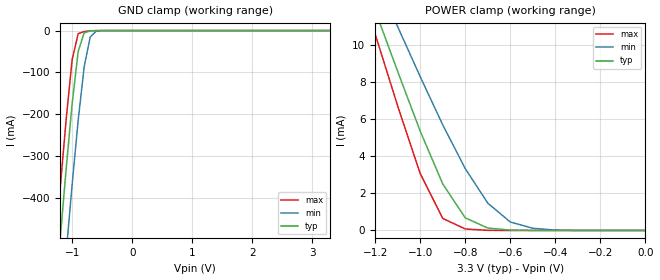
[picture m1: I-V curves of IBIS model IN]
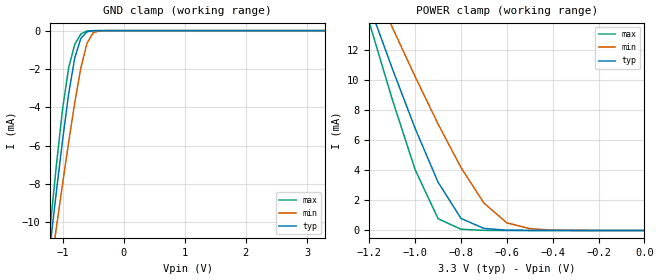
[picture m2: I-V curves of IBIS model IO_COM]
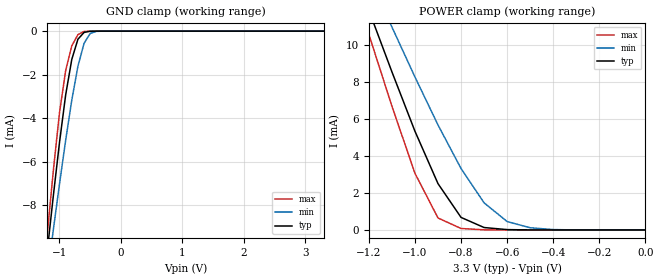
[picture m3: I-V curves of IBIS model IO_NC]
| (C) Copyright DIODES INCORPORATED
| DIODES CORPORATION
| IBIS Model of PI5A23157
| MSOP-10 (U) Package
[IBIS Ver] 3.2
[Comment char] |_char
[File Name] pi5a23157_u_33v.ibs
[File Rev] 1.0
[Source] File originated at Diodes Incorporated.
[Date] 28/11/24
[Disclaimer]
   All rights reserved
  DIODES Corporation hereby grants the user of
  this IBIS model a non-exclusive, nontransferable license to
  use this IBIS model under the following terms.
  This IBIS model is provided on an "AS IS" basis and Diodes
  makes absolutely no warranty with respect to the information
  contained herein. DIODES DISCLAIMS AND CUSTOMER WAIVES ALL
  WARRANTIES, EXPRESSED OR IMPLIED, INCLUDING WARRANTIES OF
  MERCHANTABILITY OR FITNESS FOR A PARTICULAR PURPOSE. The
  entire risk as to quality and performance is with the customer.
  Accordingly, in no event shall the company be liable for any
  damages, whether in contract or tort, including any lost
  profits or other incidental, consequential, exemplary, or
  punitive damages arising out of the use or application of the
  IBIS model provided in this package. Further, Diodes reserves
  the right to make changes without notice to any product herein
  to improve reliability, function, or design. Diodes does not
  convey any license under patent rights or any other intellectual
  property rights, including those of third parties.
  The user is granted this license only to use the IBIS model
  and is not granted rights to sell, load, rent, lease or license
  the IBIS model in whole or in part, or in modified form to anyone
  other than user. User may modify the IBIS model to suit its specific
  application but rights to derivative works and such modifications
  shall belong to Diodes.
  Diodes is not obligated to provide maintenance or support
  for the licensed IBIS model.
  Contact Diodes at ATTN: APPLICATION ENGINEERING / IBIS MODELS
  1545 Barber Lane Milpitas, CA 95035 USA.
[Component] PI5A23157
[Manufacturer] DIODES CORPORATION
[Package]
|   typ   min   max
R_pkg   50m   45m   55m
L_pkg   1.6n   1.44n   1.76n
C_pkg   0.56p   0.51p   0.62p
[Pin]   signal_name   model_name
1   IN1   IN
2   NO1   IO_NO
3   GND   GND
4   NO2   IO_NO
5   IN2   IN
6   COM2   IO_COM
7   NC2   IO_NC
8   VDD   POWER
9   NC1   IO_NC
10   COM1   IO_COM
[Series Switch Groups]
On   1 /   |NC1 to COM1
On   2 /   |NC2 to COM2
On   3 /   |NO1 to COM1
On   4 /   |NO2 to COM2
On   1 2 /
On   3 4 /
On   1 4 /
On   2 3 /
[Series Pin Mapping]   pin_2   model_name   function_table_group
9   10   SW_33   1
7   6   SW_33   2
2   10   SW_33   3
4   6   SW_33   4
[Model] SW_33
Model_type   Series_switch
Polarity   Non-Inverting
Enable  Active-High
C_comp   7.843pF   7.742pF   8.103pF
[Voltage Range]   3.3   3   3.6
[Temperature Range]   25   -40   125
[On]
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[off]
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| Models and submodels in the file (5): IN (Input), IO_COM (Terminator), IO_NC (Terminator), IO_NO (Terminator), SW_33 (Series_switch)
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[Model]   IN
Polarity   Non-Inverting
Model_type   Input
Vinl=0.99
Vinh=2.31
C_comp   1.924pF   1.924pF   1.925pF
[Voltage Range]   3.3   3   3.6
[Temperature Range]   25   -40   125
[GND Clamp Reference]   0   0   0
[POWER Clamp Reference]   3.3   3   3.6
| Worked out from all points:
|   GND clamp passes 1 mA (typ) near -0.69 V on its own axis
|   POWER clamp passes 1 mA (typ) near -0.82 V on its own axis
[GND_Clamp]
-3.3V     -4.308A    -4.479A    -4.209A
-1.3V     -672mA     -874.9mA   -551.1mA
-1.2V     -498.6mA   -701.3mA   -377.7mA
-1.1V     -330.7mA   -531.4mA   -212.2mA
-1V       -174.4mA   -367.4mA   -69.35mA
-900mV    -50.06mA   -214.6mA   -7.417mA
-800mV    -5.194mA   -86.41mA   -2.283mA
-700mV    -1.045mA   -15.38mA   -516.4uA
-600mV    -172uA     -1.514mA   -42.54uA
3.3V      120.3pA    1.119nA    118.8pA
[Power_Clamp]
|   X   TYP   MIN   MAX
-3.3V     55.62mA    47.6mA     65.56mA
-1.3V     15.1mA     16.35mA    14.33mA
-1.2V     11.86mA    13.68mA    10.58mA
-1.1V     8.568mA    10.98mA    6.71mA
-1V       5.353mA    8.288mA    3.067mA
-900mV    2.51mA     5.692mA    650.3uA
-800mV    679.9uA    3.332mA    79.57uA
-700mV    131.6uA    1.473mA    7.874uA
-600mV    19.19uA    456.4uA    573.5nA
-500mV    1.923uA    119.9uA    23.84nA
-400mV    133.2nA    20.66uA    1.87nA
0V        501.6pA    4.144nA    540.8pA
[Model]   IO_COM
Model_type   Terminator
C_comp   7.843pF   7.742pF   8.104pF
[Voltage Range]   3.3   3   3.6
[Temperature Range]   25   -40   125
[GND Clamp Reference]   0   0   0
[POWER Clamp Reference]   3.3   3   3.6
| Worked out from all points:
|   GND clamp passes 1 mA (typ) near -0.76 V on its own axis
|   POWER clamp passes 1 mA (typ) near -0.81 V on its own axis
[GND_Clamp]
-3.3V     -7.609A    -7.779A    -7.571A
-1.3V     -13.92mA   -15.37mA   -13.46mA
-1.2V     -11.14mA   -12.58mA   -10.2mA
-1.1V     -8.401mA   -10.27mA   -7.03mA
-1V       -5.746mA   -8.019mA   -4.119mA
-900mV    -3.309mA   -5.834mA   -1.944mA
-800mV    -1.431mA   -3.766mA   -721uA
-700mV    -405.9uA   -1.946mA   -175.1uA
-600mV    -64.82uA   -663.6uA   -15.81uA
-500mV    -5.832uA   -120.4uA   -626.3nA
-400mV    -349.3nA   -12.14uA   -15.06nA
3.3V      675.1pA    2.363uA    362pA
[Power_Clamp]
-3.3V     125.1mA    92.25mA    146.7mA
-1.2V     14.97mA    16.92mA    13.84mA
-1.1V     10.79mA    13.53mA    8.731mA
-1V       6.787mA    10.24mA    4.038mA
-900mV    3.213mA    7.086mA    783.6uA
-800mV    799.8uA    4.188mA    81.7uA
-700mV    136uA      1.822mA    7.986uA
-600mV    19.52uA    507.5uA    580.2nA
-500mV    1.948uA    124uA      24.16nA
-400mV    134.9nA    21.07uA    1.894nA
0V        674pA      4.416nA    715.2pA
[Model]   IO_NC
Model_type   Terminator
C_comp   2.961pF   2.904pF   3.040pF
[Voltage Range]   3.3   3   3.6
[Temperature Range]   25   -40   125
[GND Clamp Reference]   0   0   0
[POWER Clamp Reference]   3.3   3   3.6
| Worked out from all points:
|   GND clamp passes 1 mA (typ) near -0.77 V on its own axis
|   POWER clamp passes 1 mA (typ) near -0.82 V on its own axis
[GND_Clamp]
-3.3V     -3.99A     -4.042A    -4.001A
-1.2V     -10.14mA   -11.29mA   -9.373mA
-1.1V     -7.568mA   -9.128mA   -6.407mA
-1V       -5.123mA   -7.033mA   -3.758mA
-900mV    -2.941mA   -5.026mA   -1.818mA
-800mV    -1.3mA     -3.173mA   -676.3uA
-700mV    -371.8uA   -1.613mA   -161.9uA
-600mV    -59.28uA   -558.3uA   -14.42uA
-500mV    -5.325uA   -105.3uA   -563.4nA
-400mV    -316.2nA   -10.87uA   -13.45nA
3.3V      502pA      2.329uA    324.7pA
[Power_Clamp]
-3.3V     55.6mA     44.9mA     65.6mA
-1.3V     15.1mA     16.4mA     14.3mA
-1.2V     11.9mA     13.7mA     10.6mA
-1.1V     8.57mA     11mA       6.71mA
-1V       5.35mA     8.29mA     3.07mA
-900mV    2.51mA     5.69mA     650uA
-800mV    680uA      3.33mA     79.6uA
-700mV    132uA      1.47mA     7.87uA
-600mV    19.2uA     456uA      574nA
-500mV    1.92uA     120uA      23.8nA
-400mV    133nA      20.7uA     1.87nA
0V        502pA      4.14nA     541pA
